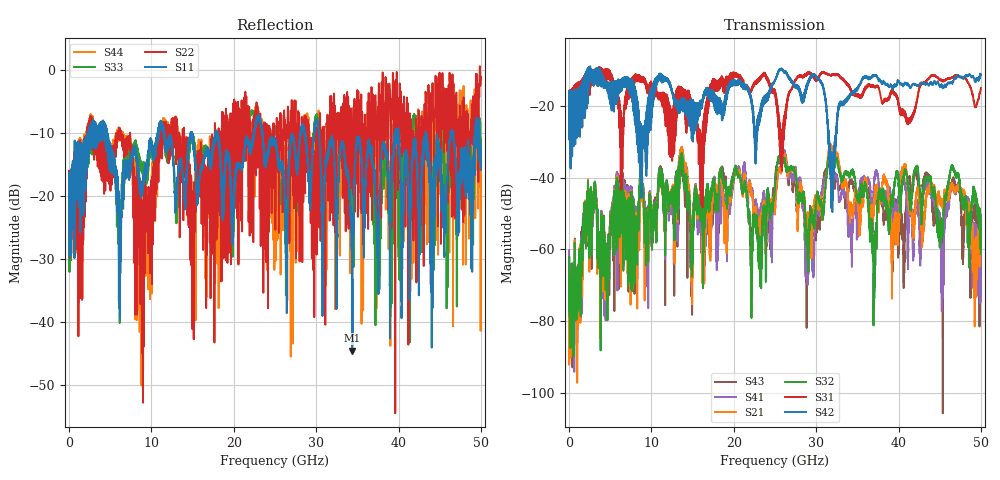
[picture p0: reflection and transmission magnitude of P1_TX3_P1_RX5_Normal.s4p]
!Keysight Technologies,N5225B,MY57041031,A.13.20.10
!Date: Friday, May 31, 2019 11:20:43
!Correction: S11(Full 4 Port(1,2,3,4))
!S12(Full 4 Port(1,2,3,4))
!S13(Full 4 Port(1,2,3,4))
!S14(Full 4 Port(1,2,3,4))
!S21(Full 4 Port(1,2,3,4))
!S22(Full 4 Port(1,2,3,4))
!S23(Full 4 Port(1,2,3,4))
!S24(Full 4 Port(1,2,3,4))
!S31(Full 4 Port(1,2,3,4))
!S32(Full 4 Port(1,2,3,4))
!S33(Full 4 Port(1,2,3,4))
!S34(Full 4 Port(1,2,3,4))
!S41(Full 4 Port(1,2,3,4))
!S42(Full 4 Port(1,2,3,4))
!S43(Full 4 Port(1,2,3,4))
!S44(Full 4 Port(1,2,3,4))
!S4P File: Measurements: <S11,S12,S13,S14>,
!<S21,S22,S23,S24>,
!<S31,S32,S33,S34>,
!<S41,S42,S43,S44>:
# Hz S  dB  R 50.0
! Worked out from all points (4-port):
!   5000 points, 10 MHz to 50 GHz, reference 50 ohm
!   strongest paths, dB at 10 MHz, 12.51 GHz, 25.01 GHz, 37.51 GHz, 50 GHz:
!     S42: -19.5, -15.6, -13.0, -12.4, -11.5
!     S31: -19.5, -27.0, -15.7, -14.5, -15.0
!     S32: -72.7, -44.5, -42.0, -47.0, -61.3
!     S21: -62.6, -43.9, -48.1, -46.3, -56.2
!     S41: -60.2, -44.8, -47.2, -40.1, -63.9
!     S43: -69.4, -45.8, -40.6, -45.9, -59.6
!   lowest |S11| = -44.5 dB at 34.39 GHz (marker M1), VSWR 1.01, Z = 50.1 + j0.588 ohm
!   |S11| at or under -10 dB: 4.66 GHz to 10.77 GHz (6.107 GHz wide, 79.2 % of centre); 23.49 GHz to 28.08 GHz (4.585 GHz wide, 17.8 % of centre); 30.37 GHz to 39.62 GHz (9.242 GHz wide, 26.4 % of centre)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
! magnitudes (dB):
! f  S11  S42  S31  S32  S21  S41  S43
! 10 MHz  -19.6  -19.5  -19.5  -72.7  -62.6  -60.2  -69.4
! 13.66 GHz  -15.0  -20.5  -19.7  -34.1  -32.4  -31.9  -34.0
! 23.18 GHz  -7.5  -24.0  -12.2  -62.0  -54.1  -51.9  -56.2
! 34.39 GHz  -44.5  -16.3  -16.2  -37.9  -49.3  -55.4  -41.6
! 37.04 GHz  -18.0  -11.4  -14.7  -64.0  -47.0  -40.8  -47.8
! 47.3 GHz  -20.6  -11.7  -11.6  -39.5  -41.8  -41.8  -42.9
! 50 GHz  -12.3  -11.5  -15.0  -61.3  -56.2  -63.9  -59.6
